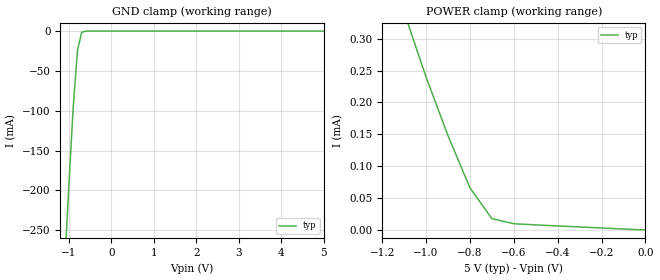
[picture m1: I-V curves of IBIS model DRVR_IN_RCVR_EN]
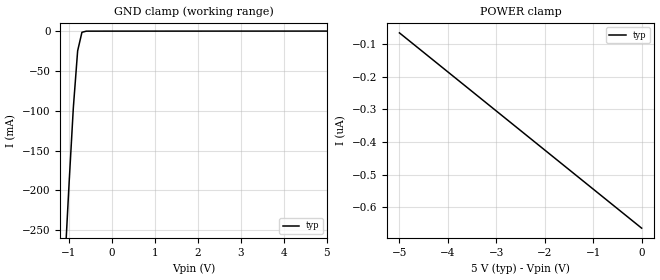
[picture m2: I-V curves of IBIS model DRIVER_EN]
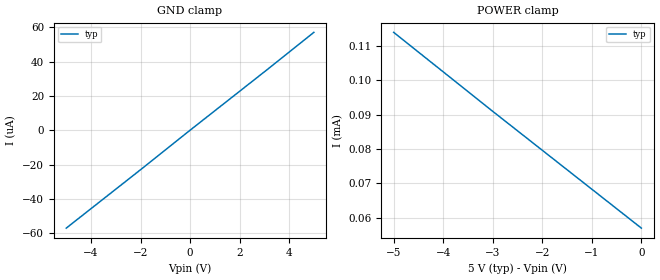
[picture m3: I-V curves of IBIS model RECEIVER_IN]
|   Texas Instruments Incorporated
|   Data Transmissions Products
|   IBIS Model for SN65LBC182
|   8D SOIC Package
[IBIS Ver]   3.2
[Comment char]   |_char
[File name]   lbc182.ibs
[File Rev]   1.0
[Date]   24May01
[Source]   File originated at Texas Instruments Incorporated.
   Data Transmission Products Group.
[Notes]
[Disclaimer]
(C) Copyright Texas Instruments Incorporated 2001
   All rights reserved
  Texas Instruments Incorporated hereby grants 1the user of this IBIS
model a non-exclusive, nontransferable license to use this IBIS model
under the following terms.  Before using this IBIS model, the user
should read this license.  If the user does not accept these terms,
the IBIS model should be returned to Texas Instruments within 30 days.
  The user is granted this license only to use the IBIS model and
is not granted rights to sell, load, rent, lease or license the IBIS
model in whole or in part, or in modified form to anyone other than
user.  User may modify the IBIS model to suit its specific applications
but rights to derivative works and such modifications shall belong to
Texas Instruments.
  This IBIS model is provided on an "AS IS" basis and Texas Instruments
makes absolutely no warranty with respect to the information contained
herein.  TEXAS INSTRUMENTS DISCLAIMS AND CUSTOMER WAIVES ALL WARRANTIES,
EXPRESS OR IMPLIED, INCLUDING WARRANTIES OF MERCHANTABILITY OR FITNESS
FOR A PARTICULAR PURPOSE. The entire risk as to quality and performance
is with the Customer. ACCORDINGLY, IN NO EVENT SHALL THE COMPANY BE LIABLE
FOR ANY DAMAGES, WHETHER IN CONTRACT OR TORT,INCLUDING ANY LOST PROFITS
OR OTHER INCIDENTAL, CONSEQUENTIAL, EXEMPLARY, OR PUNITIVE DAMAGES ARISING
OUT OF THE USE OR APPLICATION OF THE IBIS model provided in this package.
Further, Texas Instruments reserves the right to discontinue or make changes
without notice to any product herein to improve reliability, function, or
design. Texas Instruments does not convey any license under patent rights
or any other intellectual property rights, including those of third parties.
Contact Texas Instruments at ATTN:DATA TRANSMISSIONS
[Copyright]   Copyright 2001, Texas Instruments, All Rights Reserved
[Component]   65LBC182D
[Manufacturer]  Texas Instruments Incorporated
[Package]
|   typ   min   max
R_pkg   0.036   0.033   0.039
L_pkg   3.340nH   2.445nH   4.233nH
C_pkg   0.470pF   0.308pF   0.631pF
[Pin]   signal_name   model_name   R_pin   L_pin   C_pin
1   R   RECEIVER_OUT   0.034   4.233n   0.630p
2   RE   DRVR_IN_RCVR_EN   0.038   2.445n   0.309p
3   DE   DRIVER_EN   0.039   2.448n   0.309p
4   D   DRVR_IN_RCVR_EN   0.033   4.231n   0.631p
5   GND   GND   0.033   4.230n   0.630p
6   A   REC/DRVR_BI   0.039   2.450n   0.308p
7   B   REC/DRVR_BI   0.039   2.448n   0.309p
8   VCC   POWER   0.033   4.231n   0.630p
[Diff_pin]   inv_pin   vdiff   tdelay_typ   tdelay_min   tdelay_max
| The 'A' pin is Diff_pin and the 'B' pin is the inv_pin
6   7   0.200   0 0 0
| Models and submodels in the file (5): DRVR_IN_RCVR_EN (Input), DRIVER_EN (Input), RECEIVER_IN (Input), REC/DRVR_BI (I/O), RECEIVER_OUT (3-state)
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|   Driver Input MODEL
[Model]   DRVR_IN_RCVR_EN
Model_type   Input
|Signals   D,RE
Vinh = 2.0
Vinl = 0.8
|   typ   min   max
C_comp   1.0pF   NA   NA
|   typ   min   max
[Temperature Range]   25.0   NA   NA
[Voltage range]   5.0V   4.75V   5.25V
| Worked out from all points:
|   GND clamp passes 1 mA (typ) near -0.67 V on its own axis
[GND_clamp]
|   Voltage   I(typ)   I(min)   I(max)
-5V       -4.21A     NA         NA
-2V       -1.22A     NA         NA
-1V       -192mA     NA         NA
-900mV    -96.1mA    NA         NA
-800mV    -24.8mA    NA         NA
-700mV    -1.47mA    NA         NA
-500mV    -28.2uA    NA         NA
5V        11.6pA     NA         NA
[Power_clamp]
| Note that the[POWER_clamp]voltage table is referenced to Vcc
| and is calculated using Vtable=Vcc - Vmeasured.
|   Voltage   I(typ)   I(min)   I(max)
-5V       4.42mA     NA         NA
-2V       1.26mA     NA         NA
-1V       240uA      NA         NA
-900mV    148uA      NA         NA
-800mV    66.3uA     NA         NA
-700mV    17.8uA     NA         NA
-600mV    9.8uA      NA         NA
0V        11.6pA     NA         NA
|   Driver Enable  MODEL
[Model]   DRIVER_EN
Model_type   Input
|Signals   DE
Vinh = 2.0
Vinl = 0.8
|   typ   min   max
C_comp   1.0pF   NA   NA
|   typ   min   max
[Temperature Range]   25.0   NA   NA
[Voltage range]   5.0V   4.75V   5.25V
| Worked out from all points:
|   GND clamp passes 1 mA (typ) near -0.67 V on its own axis
[GND_clamp]
|   Voltage   I(typ)   I(min)   I(max)
-5V       -4.21A     NA         NA
-2V       -1.22A     NA         NA
-1V       -192mA     NA         NA
-900mV    -96.1mA    NA         NA
-800mV    -24.8mA    NA         NA
-700mV    -1.47mA    NA         NA
-500mV    -17.2uA    NA         NA
5V        57.8uA     NA         NA
[Power_clamp]
| Note that the[POWER_clamp]voltage table is referenced to Vcc
| and is calculated using Vtable=Vcc - Vmeasured.
|   Voltage   I(typ)   I(min)   I(max)
-5V       -66.4nA    NA         NA
0V        -664nA     NA         NA
|   Receiver Input MODEL
[Model]   RECEIVER_IN
Model_type   Input
|Signals   A,B
Vinl = 2.1V
Vinh = 2.5V
|   typ   min   max
C_comp   1.0pF   NA   NA
|   typ   min   max
[Temperature Range]   25.0   NA   NA
[Voltage range]   5.0V   4.75V   5.25V
[GND_clamp]
|   Voltage   I(typ)   I(min)   I(max)
-5V       -57uA      NA         NA
-2V       -23uA      NA         NA
0V        0A         NA         NA
3V        34uA       NA         NA
5V        57uA       NA         NA
[Power_clamp]
| Note that the[POWER_clamp]voltage table is referenced to Vcc
| and is calculated using Vtable=Vcc - Vmeasured.
|   Voltage   I(typ)   I(min)   I(max)
-5V       114uA      NA         NA
-3V       91uA       NA         NA
0V        57uA       NA         NA
